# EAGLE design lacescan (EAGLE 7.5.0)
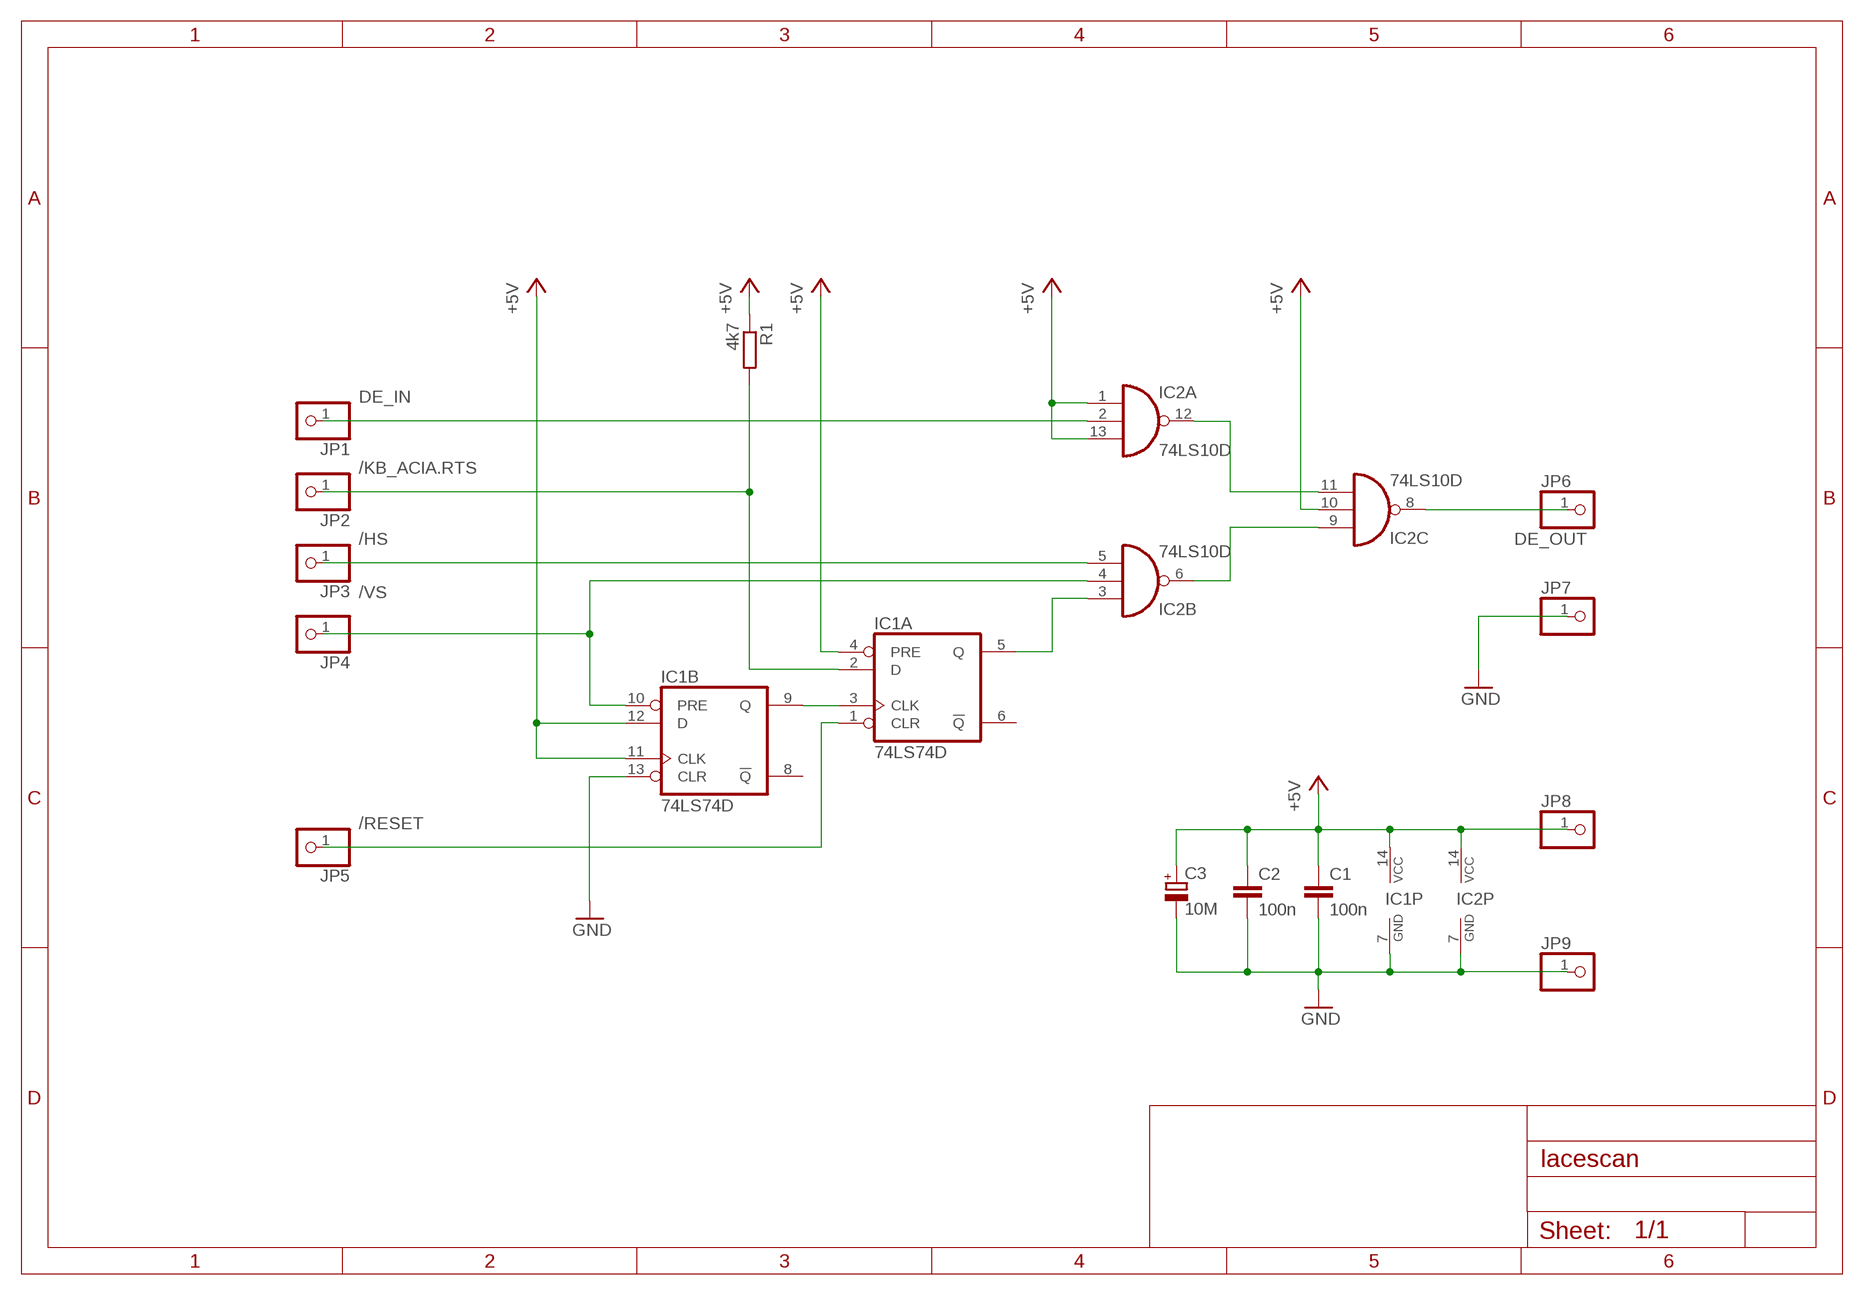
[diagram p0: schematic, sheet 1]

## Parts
C1  100n  C-EUC0805  [C0805]
C2  100n  C-EUC0805  [C0805]
C3  10M  CPOL-EUA/3216-18R  [A/3216-18R]
IC1  74LS74D  [SO14]
IC2  74LS10D  [SO14]
JP1  PINHD-1X1  [1X01]
JP2  PINHD-1X1  [1X01]
JP3  PINHD-1X1  [1X01]
JP4  PINHD-1X1  [1X01]
JP5  PINHD-1X1  [1X01]
JP6  PINHD-1X1  [1X01]
JP7  PINHD-1X1  [1X01]
JP8  PINHD-1X1  [1X01]
JP9  PINHD-1X1  [1X01]
R1  4k7  R-EU_M0805  [M0805]

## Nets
+5V: C1.1 C2.1 C3.+ IC1.4(A:PRE) IC1.11(B:CLK) IC1.12(B:D) IC1.14(P:VCC) IC2.1(A:I0) IC2.10(C:I1) IC2.13(A:I2) IC2.14(P:VCC) JP8.1 R1.1
/HS: IC2.5(B:I2) JP3.1
/KB_ACIA.RTS: IC1.2(A:D) JP2.1 R1.2
/RESET: IC1.1(A:CLR) JP5.1
/VS: IC1.10(B:PRE) IC2.4(B:I1) JP4.1
DE_IN: IC2.2(A:I1) JP1.1
DE_OUT: IC2.8(C:O) JP6.1
GND: C1.2 C2.2 C3.- IC1.7(P:GND) IC1.13(B:CLR) IC2.7(P:GND) JP7.1 JP9.1
N$1: IC1.3(A:CLK) IC1.9(B:Q)
N$2: IC1.5(A:Q) IC2.3(B:I0)
N$3: IC2.6(B:O) IC2.9(C:I0)
N$4: IC2.11(C:I2) IC2.12(A:O)
Unconnected: IC1.6(A:!Q) IC1.8(B:!Q)

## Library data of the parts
C1 C2 = rcl:C-EU: CAPACITOR, European symbol
C3 = rcl:CPOL-EU: POLARIZED CAPACITOR, European symbol
IC1 = 74xx-eu:74*74: Dual D type positive edge triggered FLIP FLOP, preset and clear
IC2 = 74xx-eu:74*10: Triple 3-input NAND gate
JP1-JP9 = pinhead:PINHD-1X1: PIN HEADER
R1 = rcl:R-EU_: RESISTOR, European symbol

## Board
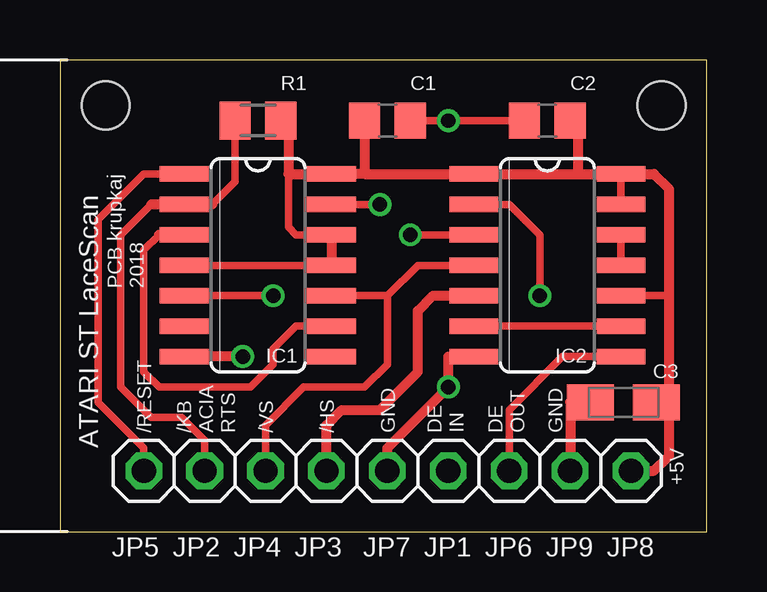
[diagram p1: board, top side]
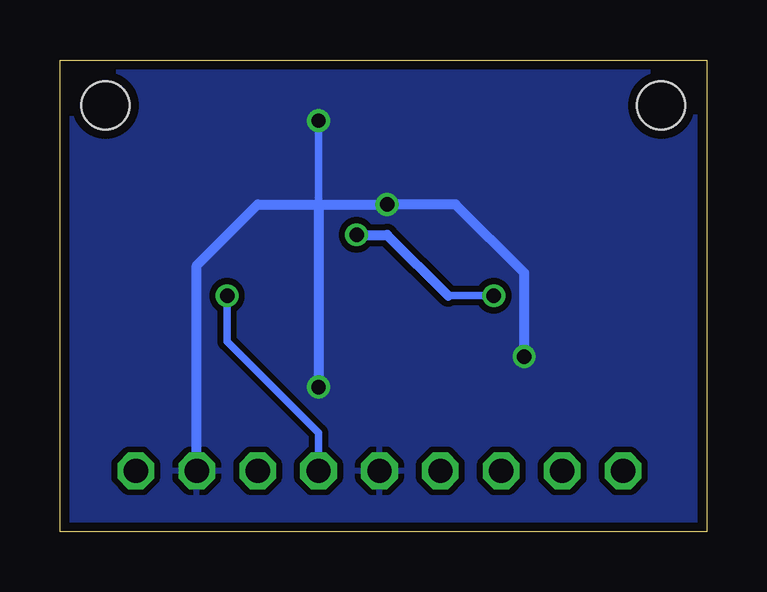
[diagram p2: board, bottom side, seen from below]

Size 26.98 x 19.68 mm. Coordinates in mm from the lower left corner, seen from the top.
Outline: 0,0 26.98,0 26.98,19.68 0,19.68 0,0
Copper layers (1*16): Top 0.0356mm / dielectric 1.5011mm / Bottom 0.0356mm
Design rules "OSH_Park_LaenPCBOrder": minimum track width 6mil, minimum drill 13mil, track to track 6mil, track to pad 6mil, pad to pad 6mil, via to via 6mil, smd to smd 6mil, copper to edge 15mil, drill to drill 6mil, minimum pad ring 7mil, minimum via ring 7mil, stop-mask expansion 3mil, vias tented up to drill 0mil, thermal gap 10mil
Holes 2 mm at 1.91,17.78 25.08,17.78

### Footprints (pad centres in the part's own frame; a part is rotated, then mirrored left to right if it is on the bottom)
C0805 = smd 1.3 x 1.5: 1 -0.95,0; 2 0.95,0
A/3216-18R = smd 1.95 x 1.5: + 1.375,0; - -1.375,0
SO14 = smd 0.66 x 2.032: 1 -3.81,-3.073; 2 -2.54,-3.073; 3 -1.27,-3.073; 4 0,-3.073; 5 1.27,-3.073; 6 2.54,-3.073; 7 3.81,-3.073; 8 3.81,3.073; 9 2.54,3.073; 10 1.27,3.073; 11 0,3.073; 12 -1.27,3.073; 13 -2.54,3.073; 14 -3.81,3.073
1X01 = drill 1.016 octagon: 1 0,0
M0805 = smd 1.3 x 1.6: 1 -0.95,0; 2 0.95,0

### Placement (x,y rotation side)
C1  13.65,17.15 0 top
C2  20.32,17.15 180 top
C3  23.49,5.4 0 top
IC1  8.26,11.11 270 top
IC2  20.32,11.11 270 top
JP1  16.19,2.54 270 top
JP2  6.03,2.54 0 top
JP3  11.11,2.54 0 top
JP4  8.57,2.54 0 top
JP5  3.49,2.54 0 top
JP6  18.73,2.54 0 top
JP7  13.65,2.54 0 top
JP8  23.81,2.54 0 top
JP9  21.27,2.54 0 top
R1  8.26,17.15 180 top

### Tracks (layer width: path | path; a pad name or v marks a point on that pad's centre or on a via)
+5V
  Top 0.305: 21.59,14.92 22.86,14.93 | C1.1 | IC1.11 IC1.4 | IC1.14 12.38,14.92 12.7,14.92 | IC1.12 9.84,12.38 9.52,12.7 9.52,14.92 | IC2.13 IC2.14 | IC2.10 25.4,9.84
  Top 0.406: 21.59,16.83 21.59,14.92 | IC1.11 IC1.12 11.43,12.38 | C1.1 12.7,14.92 | 12.7,14.92 12.38,14.93 12.38,14.92 | R1.1 9.52,16.83 9.52,14.92 IC1.14 | 12.7,14.92 IC2.1 21.59,14.92 | 21.59,14.92 24.77,14.92 25.4,14.29 25.4,9.84 25.4,5.08 25.4,3.17 24.77,2.54 JP8.1
  Top 0.61: C2.1 21.59,16.83 | 22.86,14.93 22.54,14.92 IC2.14 | C3.+ 25.4,5.08
/HS
  Top 0.406: JP3.1 11.11,4.44 11.75,5.08 13.34,5.08 14.92,6.67 14.92,9.21 15.56,9.84 IC2.5
/KB_ACIA.RTS
  Top 0.305: 3.81,13.65 2.54,12.38 2.54,6.03 3.81,4.76 5.08,4.76 6.03,3.81 JP2.1 | R1.2 7.3,14.6 6.35,13.65
  Top 0.406: 3.81,13.65 IC1.2 6.35,13.65
/RESET
  Top 0.305: IC1.1 3.49,14.92 1.59,13.02 1.59,5.4 3.49,3.49 JP5.1
/VS
  Top 0.305: JP4.1 8.57,4.44 10.16,6.03 12.7,6.03 13.65,6.98 13.65,9.84 | 13.65,9.84 14.92,11.11 IC2.4 | IC1.10 13.65,9.84
DE_IN  (via drill 0.6)
  Top 0.305: IC2.2 18.73,13.65 20,12.38 v20,9.84
  Bottom 0.305: v20,9.84 20,7.94 16.19,4.13 JP1.1
DE_OUT
  Top 0.305: IC2.8 20.95,7.3 18.73,5.08 JP6.1
GND  (via drill 0.6)
  Top 0.305: C2.2 v16.19,17.15 C1.2 | v13.34,13.65 IC1.13
  Top 0.406: v7.62,7.3 IC1.7 | IC2.7 16.19,7.3 v16.19,6.03 13.65,3.49 JP7.1 | C3.- 21.27,5.4 JP9.1
  Bottom 0.305: v16.19,17.15 16.19,13.65
  Bottom 0.406: v13.34,13.65 10.48,13.65 7.62,10.8 v7.62,7.3 | v16.19,6.03 16.19,13.65 v13.34,13.65 | JP9.1 21.27,11.11 18.73,13.65 v13.34,13.65
  pour Bottom (isolate 0.254): -1.91,22.23 -1.91,-2.86 29.21,-2.86 29.21,22.23
N$1
  Top 0.305: 4.13,12.38 3.49,11.75 3.49,6.67 4.13,6.03 7.94,6.03 8.89,6.98 8.89,7.62 9.84,8.57 IC1.9
  Top 0.406: IC1.3 4.13,12.38
N$2  (via drill 0.6)
  Top 0.305: IC2.3 v14.6,12.38 | IC1.5 v8.89,9.84
  Bottom 0.305: 10.8,9.84 v8.89,9.84
  Bottom 0.406: v14.6,12.38 13.34,12.38 10.8,9.84
N$3
  Top 0.305: IC2.6 IC2.9
N$4
  Top 0.305: IC2.12 IC2.11

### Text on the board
tNames: PCB krupkaj / 2018 | /RESET | /KB / ACIA / RTS | /VS | /HS | GND | DE / IN | DE / OUT | GND | ATARI ST LaceScan | +5V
